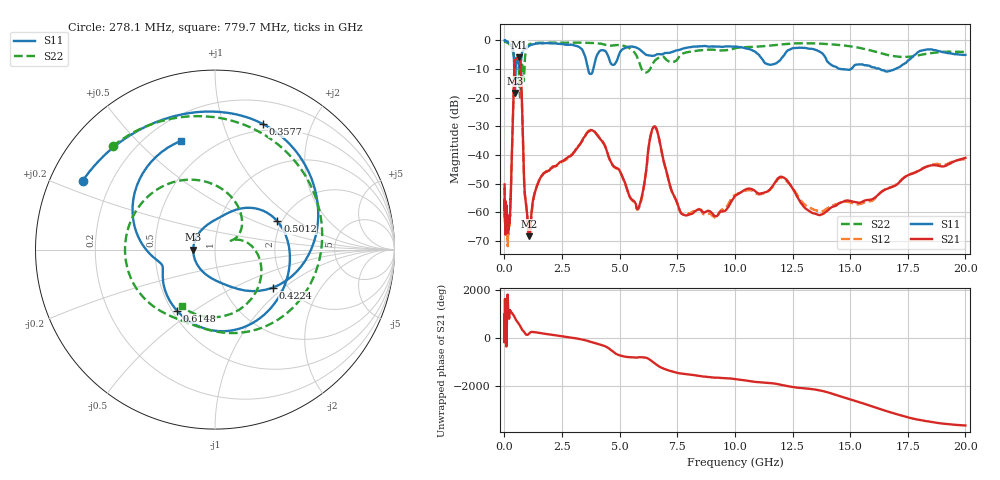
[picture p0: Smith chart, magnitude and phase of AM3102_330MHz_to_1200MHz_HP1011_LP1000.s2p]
! Date/Time: Tue, Sep 11, 2018 5:20 PM
! Network Analyzer: Agilent Technologies E8362B Rev: A.07.50.63
! Sweep from 0.010 to 20.000 GHz, 1601 Points, Sweep Type: LOG
! Power Supply: 4.949 V, 0.001 A
# Hz S DB R 50
!freq MagS11 AngS11 MagS21 AngS21 MagS12 AngS12 MagS22 AngS22
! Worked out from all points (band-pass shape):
!   1601 points, 10 MHz to 20 GHz, reference 50 ohm
!   highest |S21| = -5.89 dB at 620.7 MHz (marker M1); lowest = -68.4 dB at 1.077 GHz (marker M2)
!   |S21| within 3 dB of the highest: 438.5 MHz to 700.7 MHz (262.1 MHz wide, 46 % of centre)
!   lowest |S11| = -18.3 dB at 453.6 MHz (marker M3), VSWR 1.28, Z = 39.2 - j0.0375 ohm
!   |S11| at or under -10 dB: 3.625 GHz to 3.856 GHz (231.5 MHz wide, 6.19 % of centre); 14.62 GHz to 15.03 GHz (415.8 MHz wide, 2.8 % of centre); 16.29 GHz to 16.95 GHz (659.4 MHz wide, 3.97 % of centre)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
!   |S22| runs from -19.9 to -0.2 dB; largest |S21 - S12| = 0.0094
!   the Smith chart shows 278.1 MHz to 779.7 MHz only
!   S11 on the Smith chart (normalised r, x): 278.1 MHz: 0.10, +0.24; 357.7 MHz: 0.43, +1.36; 422.4 MHz: 1.69, -0.84; 501.2 MHz: 1.90, +0.70; 614.8 MHz: 0.53, -0.43; 779.7 MHz: 0.33, +0.68
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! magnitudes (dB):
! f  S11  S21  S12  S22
! 10 MHz  0.0  -50.3  -52.2  -0.2
! 35.55 MHz  0.0  -65.2  -65.3  -0.4
! 126.4 MHz  -0.4  -65.4  -63.0  -0.8
! 278.1 MHz  -1.6  -54.1  -53.6  -1.8
! 357.7 MHz  -2.5  -29.3  -29.4  -3.6
! 422.4 MHz  -8.3  -11.4  -11.5  -6.1
! 447.2 MHz  -17.7  -8.0  -8.0  -7.1
! 453.6 MHz  -18.3  -7.5  -7.5  -7.2
! 501.2 MHz  -8.4  -6.5  -6.5  -6.2
! 614.8 MHz  -7.9  -5.9  -6.0  -9.5
! 620.7 MHz  -8.2  -5.9  -6.0  -10.2
! 779.7 MHz  -3.9  -26.6  -26.7  -8.7
! 873.8 MHz  -3.1  -52.1  -52.4  -9.3
! 1.077 GHz  -1.9  -68.4  -69.1  -1.4
! 1.59 GHz  -1.0  -47.6  -47.5  -0.8
! 3.811 GHz  -11.2  -31.4  -31.3  -0.9
! 5.652 GHz  -2.3  -56.4  -56.7  -4.3
! 6.518 GHz  -5.3  -30.0  -30.2  -7.1
! 7.92 GHz  -2.5  -61.1  -60.7  -4.1
! 12.03 GHz  -6.2  -47.7  -48.0  -1.4
! 13.74 GHz  -4.2  -60.8  -59.8  -1.1
! 20 GHz  -5.0  -41.0  -41.4  -4.0
